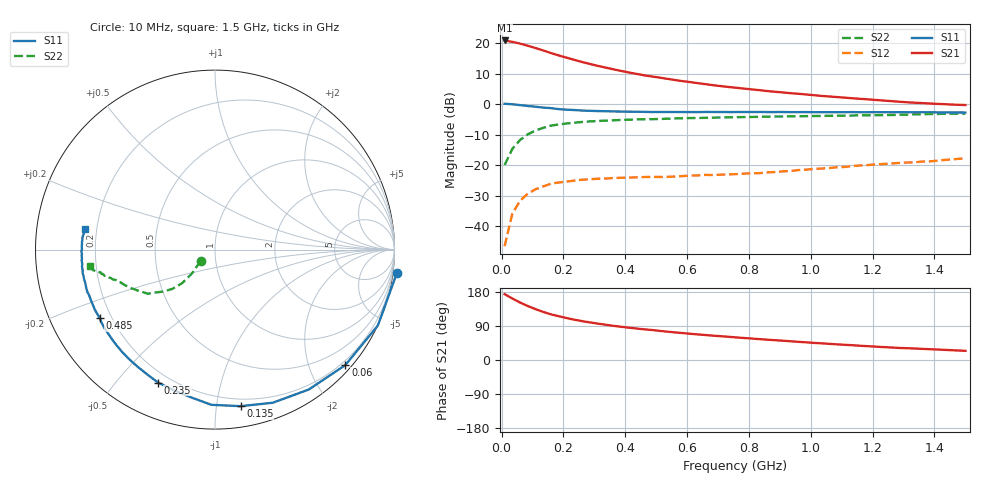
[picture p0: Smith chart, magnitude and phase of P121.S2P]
! Date: ! Date: Fri Jun 07 10:40:46 1996
# MHZ  S  MA  R  50.0000
!  POLYFET RF DEVICES
!  P121
!  S PARAMETERS
!  VDS=12.5V, IDQ=250mA
!FREQ  S11MAG S11ANG S21MAG S21ANG S12MAG S12ANG S22MAG S22ANG
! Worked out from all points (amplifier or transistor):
!   61 points, 10 MHz to 1.5 GHz, reference 50 ohm
!   highest |S21| = 20.9 dB at 10 MHz (marker M1)
!   |S21| within 3 dB of that: start of sweep to 126.1 MHz
!   unconditionally stable (mu >= 1): nowhere
!   at 260 MHz: K = 0.37, MSG = 19.3 dB, |S12| = -24.7 dB
!   at 760 MHz: K = 0.89, MSG = 14.1 dB, |S12| = -22.9 dB
!   at 1.5 GHz: K = 0.77, MSG = 8.7 dB, |S12| = -17.6 dB
!   S11 on the Smith chart (normalised r, x): 10 MHz: -3, -15; 60 MHz: 0.12, -2.63; 135 MHz: 0.15, -1.17; 235 MHz: 0.15, -0.65; 485 MHz: 0.16, -0.27; 1.5 GHz: 0.16, +0.08
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10  1.022 -7.3  11.13 173.9  0.00473 78.0  0.1011 -141.8
35  1.001 -25.0  10.55 162.2  0.01614 73.9  0.186 -133.9
60  0.9701 -41.5  9.876 151.7  0.02624 65.5  0.2602 -134.3
85  0.9387 -56.1  9.12 142.3  0.03435 58.9  0.3222 -137.3
110  0.912 -69.3  8.354 134.2  0.04046 52.7  0.3727 -141.1
135  0.8838 -80.7  7.624 126.9  0.04514 48.0  0.4112 -144.4
160  0.865 -91.3  6.907 120.4  0.04999 45.3  0.4472 -146.7
185  0.8337 -99.3  6.323 115.6  0.05233 40.2  0.4675 -149.6
210  0.8162 -106.7  5.812 110.7  0.05418 37.6  0.4846 -151.7
235  0.8059 -113.2  5.362 106.4  0.05604 35.9  0.4985 -153.6
260  0.7908 -118.8  4.941 102.7  0.05803 34.0  0.5134 -155.2
310  0.7755 -128.1  4.282 96.2  0.06026 31.4  0.5323 -157.6
360  0.765 -135.8  3.763 90.4  0.06177 29.7  0.5473 -159.5
410  0.7572 -142.0  3.336 85.4  0.06289 28.9  0.5588 -161.0
485  0.7472 -149.4  2.859 79.3  0.06459 28.2  0.5705 -162.5
510  0.7474 -151.3  2.745 77.0  0.06441 28.8  0.5736 -162.6
635  0.7459 -160.0  2.221 67.5  0.06834 30.3  0.597 -164.2
760  0.7471 -166.5  1.864 59.5  0.07183 32.3  0.6159 -165.5
860  0.7462 -171.0  1.648 53.6  0.07663 34.7  0.6263 -166.6
1010  0.7429 -176.1  1.411 45.1  0.08733 38.2  0.6427 -167.9
1260  0.7415 177.4  1.128 33.0  0.1068 38.7  0.6669 -169.8
1500  0.7326 171.1  0.9733 24.2  0.1313 41.2  0.7048 -172.5
